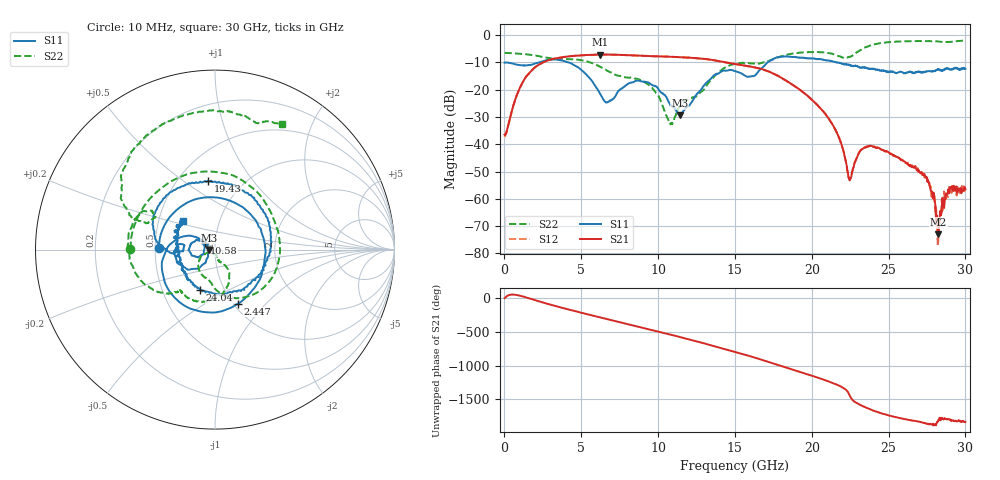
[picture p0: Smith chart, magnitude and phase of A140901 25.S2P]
!  2-Port S-parameters saved by WinCal
! VAR MeasName=S-Parameters (CALIBRATED_DATA) read from VNA (N5244A)
! VAR MeasDate=11/3/2014 9:28:54 AM
! VAR NAME=A140901 25
! VAR FILENAME=A140901 25.S2P
! VAR DATE=11/3/2014 9:28:54 AM
! VAR PHYS_PORTS=1,2
# Hz S RI R 50
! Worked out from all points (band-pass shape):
!   801 points, 10 MHz to 30 GHz, reference 50 ohm
!   highest |S21| = -7.14 dB at 6.233 GHz (marker M1); lowest = -73.0 dB at 28.24 GHz (marker M2)
!   |S21| within 3 dB of the highest: 2.472 GHz to 14.53 GHz (12.06 GHz wide, 142 % of centre)
!   lowest |S11| = -29.3 dB at 11.41 GHz (marker M3), VSWR 1.07, Z = 46.7 - j0.188 ohm
!   |S11| at or under -10 dB: start of sweep to 2.281 GHz; 4.136 GHz to 17.14 GHz (13 GHz wide, 122 % of centre); 21.65 GHz to end of sweep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
!   |S22| runs from -32.7 to -2.0 dB; largest |S21 - S12| = 0.0029
!   S11 on the Smith chart (normalised r, x): 10 MHz: 0.52, +0.01; 2.447 GHz: 1.05, -0.71; 10.58 GHz: 0.89, +0.06; 19.43 GHz: 0.70, +0.62; 24.04 GHz: 0.77, -0.37; 30 GHz: 0.67, +0.23
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1e7  -0.3117 0.00689  0.015 0.00126  0.0137 0.000599  -0.4712 0.00417
7.972375e8  0.0585 0.2805  0.0499 0.0602  0.0499 0.0602  -0.3288 0.3171
2.446688e9  0.1289 -0.3009  0.1695 -0.2575  0.1697 -0.2572  0.2243 0.3292
5.033325e9  -0.2189 0.0537  -0.3498 0.2429  -0.3489 0.2432  0.2728 -0.2101
6.232925e9  -0.0716 0.0431  0.097 0.4285  0.0967 0.4278  0.0515 -0.256
7.844888e9  -0.1087 -0.0387  0.4183 -0.0949  0.4175 -0.0944  -0.0386 -0.1631
1.001916e10  -0.0899 0.0505  -0.2785 -0.2972  -0.278 -0.2967  -0.0708 -0.0308
1.058148e10  -0.0583 0.036  -0.3887 -0.1044  -0.3887 -0.1044  -0.0258 -0.0176
1.14062e10  -0.0341 -0.00201  -0.3309 0.2118  -0.3303 0.212  0.0198 -0.0457
1.346801e10  -0.1221 -0.1076  0.3247 0.1332  0.3247 0.1322  0.0807 -0.1298
1.5005e10  -0.2179 0.00967  0.0824 -0.2829  0.0802 -0.2817  -0.0587 -0.2909
1.65045e10  -0.209 -0.0141  -0.2456 -0.0255  -0.2457 -0.0251  -0.1918 -0.2304
1.942852e10  -0.038 0.3811  0.0812 -0.0392  0.081 -0.0381  -0.475 -0.0461
2.002832e10  0.0931 0.3632  0.0222 -0.0605  0.0229 -0.0604  -0.4825 0.0455
2.156531e10  0.3103 0.0614  -0.0172 0.00443  -0.0173 0.00426  -0.3686 0.2142
2.246501e10  0.2365 -0.1506  0.00218 8.84e-05  0.00221 0.000256  -0.37 0.1533
2.403949e10  -0.0844 -0.2259  -0.00591 0.00687  -0.00601 0.00677  -0.5188 0.4277
2.501416e10  -0.1671 -0.123  0.00333 0.00625  0.00331 0.00617  -0.3858 0.6328
2.737588e10  -0.2125 0.0231  0.00171 -0.00197  0.00146 -0.002  0.0519 0.7701
2.823809e10  -0.2217 0.0638  0.000224 -1.72e-05  0.000158 -7.33e-05  0.1768 0.7377
2.902532e10  -0.2095 0.103  0.00164 2.86e-05  0.00155 -0.000231  0.2461 0.7058
3e10  -0.179 0.1601  0.00122 -0.000861  0.00112 -0.000959  0.3731 0.6996
